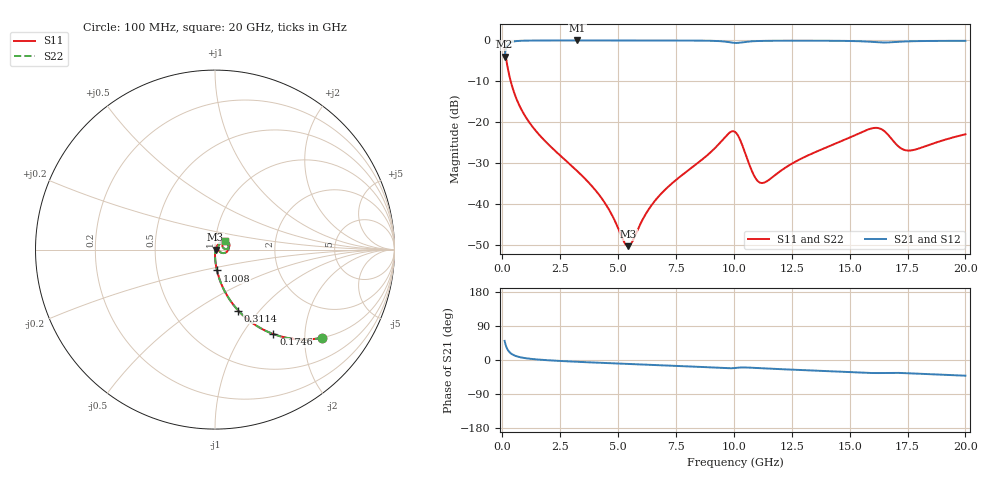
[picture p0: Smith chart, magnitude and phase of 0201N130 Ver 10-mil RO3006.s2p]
# GHz S MA R 50
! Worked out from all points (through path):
!   1601 points, 100 MHz to 20 GHz, reference 50 ohm
!   highest |S21| = -0.02 dB at 3.247 GHz (marker M1); lowest = -4.0 dB at 100 MHz (marker M2)
!   group delay of S21, straight-line fit = 6.67 ps
!   lowest |S11| = -50.2 dB at 5.436 GHz (marker M3), VSWR 1.01, Z = 50.3 - j0.0661 ohm
!   |S11| at or under -10 dB: 364.6 MHz to end of sweep
!   |S22| runs from -50.2 to -2.2 dB; largest |S21 - S12| = 0
!   S11 on the Smith chart (normalised r, x): 100 MHz: 0.99, -2.43; 174.6 MHz: 0.99, -1.39; 311.4 MHz: 0.99, -0.78; 1.008 GHz: 0.99, -0.23; 20 GHz: 1.11, +0.10
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0.1  0.7733 -39.5  0.6334 50.5  0.6334 50.5  0.7733 -39.5
0.174625  0.5723 -55.3  0.8191 34.6  0.8191 34.6  0.5723 -55.3
0.3114375  0.3638 -69.1  0.9305 20.7  0.9305 20.7  0.3638 -69.1
0.5975  0.198 -79.4  0.9791 10.3  0.9791 10.3  0.198 -79.4
1.007937  0.1165 -84.6  0.9919 4.8  0.9919 4.8  0.1165 -84.6
1.766625  0.06233 -88.3  0.9963 0.2  0.9963 0.2  0.06233 -88.3
3.246688  0.02523 -89.6  0.9973 -4.8  0.9973 -4.8  0.02523 -89.6
3.420812  0.02262 -89.3  0.9973 -5.3  0.9973 -5.3  0.02262 -89.3
4.415813  0.01053 -83.0  0.9971 -7.9  0.9971 -7.9  0.01053 -83.0
5.435688  0.00308 -12.3  0.9968 -10.4  0.9968 -10.4  0.00308 -12.3
6.741625  0.01236 58.9  0.996 -13.6  0.996 -13.6  0.01236 58.9
9.776375  0.07326 29.6  0.9525 -21.9  0.9525 -21.9  0.07326 29.6
10.05  0.07638 4.4  0.9302 -21.0  0.9302 -21.0  0.07638 4.4
10.27388  0.06087 -16.2  0.939 -19.8  0.939 -19.8  0.06087 -16.2
10.85844  0.02277 -16.3  0.977 -20.7  0.977 -20.7  0.02277 -16.3
11.15694  0.01825 6.7  0.9836 -21.7  0.9836 -21.7  0.01825 6.7
13.37081  0.04148 50.5  0.9903 -27.6  0.9903 -27.6  0.04148 50.5
15.95781  0.08435 28.4  0.9581 -34.4  0.9581 -34.4  0.08435 28.4
16.69162  0.06887 4.2  0.9444 -33.8  0.9444 -33.8  0.06887 4.2
17.17669  0.04903 8.6  0.963 -34.2  0.963 -34.2  0.04903 8.6
17.56225  0.04519 20.8  0.9735 -35.1  0.9735 -35.1  0.04519 20.8
20  0.07147 40.5  0.9869 -41.4  0.9869 -41.4  0.07147 40.5
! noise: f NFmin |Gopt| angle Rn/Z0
0.1  0.0006557  0.9345  0.3525  0.002231
2.301  0.004163  0.7813  4.49  0.003898
4.515  0.00698  0.7492  8.666  0.005573
6.729  0.009936  0.7397  12.83  0.00755
8.943  0.01897  0.812  16.99  0.0206
11.14  0.02657  0.8318  21.16  0.03221
13.36  0.02101  0.7571  25.19  0.01668
15.57  0.03868  0.8401  29.28  0.04799
17.79  0.03822  0.8187  33.31  0.04056
20  0.02783  0.7352  37.13  0.01892
